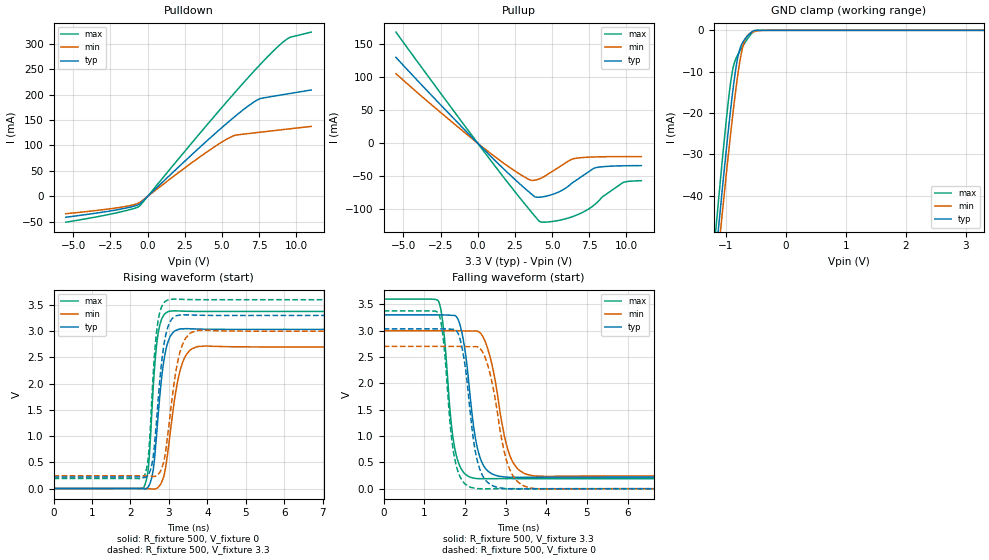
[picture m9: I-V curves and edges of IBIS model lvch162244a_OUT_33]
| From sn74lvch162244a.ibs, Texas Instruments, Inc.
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[Model]   lvch162244a_OUT_33
Model_type  3-state
Enable   Active-Low
Vref =   0
Rref =   500
Cref =   50p
Vmeas =   1.5
| variable   typ   min   max
C_comp   4.77pF   4.07pF   5.92pF
| C_pullup   2.94pF   2.22pF   4.55pF
| C_pulldown   2.77pF   2.29pF   3.86pF
| C_tri-state   4.77pF   4.07pF   5.92pF
[Temperature Range]   40   100   -40
| Ambient temperature   25   85   -40
[Voltage range]   3.3   3   3.6
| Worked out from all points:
|   slope of the pulldown table from 0 to 0.495 V, typ, clamps not added: 35.7 ohm
|   slope of the pullup table from 0 to 0.495 V, typ, clamps not added: 43.8 ohm
|   GND clamp passes 1 mA (typ) near -0.61 V on its own axis
|   rising waveform, R_fixture 500, V_fixture 0: 20-80 % time 236ps typ, 319ps min, 179ps max; typ from 0 V to 3.03 V
|   falling waveform, R_fixture 500, V_fixture 3.3: 20-80 % time 298ps typ, 400ps min, 236ps max; typ from 3.3 V to 0.22 V
|   rising waveform, R_fixture 500, V_fixture 3.3: 20-80 % time 234ps typ, 308ps min, 176ps max; typ from 0.22 V to 3.3 V
|   falling waveform, R_fixture 500, V_fixture 0: 20-80 % time 297ps typ, 396ps min, 237ps max; typ from 3.04 V to 0 V
[GND Clamp]
| lvch162244a_OUT_33
|   Voltage   I(typ)   I(min)   I(max)
-5.5V     -768.1mA   -753.5mA   -792mA
-1.18V    -56.86mA   -62.13mA   -50.54mA
-1.15V    -52.28mA   -57.69mA   -45.76mA
-1.1V     -44.75mA   -50.35mA   -37.9mA
-1.075V   -41.03mA   -46.73mA   -34.04mA
-955mV    -23.91mA   -29.87mA   -16.84mA
-885mV    -14.93mA   -20.68mA   -9.567mA
-810mV    -7.325mA   -11.87mA   -6.191mA
-745mV    -3.716mA   -5.877mA   -4.504mA
-610mV    -937.7uA   -884.1uA   -1.502mA
-470mV    -8.737uA   -130.2uA   -12.48uA
3.3V      64.68pA    54.59nA    -2.347nA
[Pulldown]
| lvch162244a_OUT_33
|   Voltage   I(typ)   I(min)   I(max)
-5.5V     -40.97mA   -34.05mA   -50.7mA
-1.905V   -25.55mA   -21.78mA   -31.11mA
-545mV    -15.11mA   -12.05mA   -19.05mA
2.915V    80.44mA    64.9mA     103.1mA
5.015V    135.8mA    107.1mA    175.4mA
5.895V    157.6mA    120.2mA    205mA
7.085V    184.2mA    124.5mA    243.9mA
7.645V    192.8mA    126.4mA    261.5mA
8.665V    197.8mA    129.8mA    291.7mA
9.36V     201.2mA    132.1mA    308.9mA
9.625V    202.5mA    133mA      313mA
11V       209.1mA    137.5mA    322.8mA
[Pullup]
| lvch162244a_OUT_33
|   Voltage   I(typ)   I(min)   I(max)
-5.5V     130.3mA    105.5mA    168.7mA
-1.46V    33.96mA    27.14mA    44.29mA
1.58V     -35.43mA   -27.59mA   -46.97mA
3.45V     -74.05mA   -55.08mA   -100.1mA
3.84V     -81.3mA    -56.09mA   -110.8mA
4.145V    -81.92mA   -54.11mA   -118.5mA
5.41V     -74.33mA   -37.07mA   -117.3mA
6.47V     -58.44mA   -23.37mA   -110.6mA
7.93V     -37.15mA   -20.8mA    -91.9mA
8.355V    -35.73mA   -20.57mA   -81.85mA
9.75V     -34.25mA   -20.26mA   -59.96mA
11V       -34.01mA   -20.24mA   -56.83mA
[Ramp]
| lvch162244a_OUT_33
| variable   typ   min   max
dV/dt_r   1.83/2.46E-10   1.63/3.32E-10   2.03/1.82E-10
dV/dt_f   1.85/3.08E-10   1.66/4.10E-10   2.05/2.40E-10
R_load = 500
[Rising Waveform]
| lvch162244a_OUT_33
R_fixture =   500
C_fixture =   0
L_fixture =   0
V_fixture =   0
V_fixture_min = 0
V_fixture_max = 0
|   Time   V(typ)   V(min)   V(max)
0s        711.3pV    1.74nV     18.52nV
2.34ns    -5.624mV   153.9uV    14.28mV
2.47ns    41.8mV     -3.632mV   423.2mV
2.595ns   368.6mV    -11.87mV   1.956V
2.71ns    1.302V     16.22mV    2.907V
2.86ns    2.391V     214mV      3.297V
3.03ns    2.894V     1.036V     3.382V
3.33ns    3.045V     2.346V     3.383V
3.8ns     3.039V     2.711V     3.376V
40ns      3.034V     2.7V       3.376V
[Falling Waveform]
| lvch162244a_OUT_33
R_fixture =   500
C_fixture =   0
L_fixture =   0
V_fixture =   3.3
V_fixture_min = 3
V_fixture_max = 3.6
|   Time   V(typ)   V(min)   V(max)
0s        3.3V       3V         3.6V
1.345ns   3.3V       3V         3.566V
1.47ns    3.298V     3V         3.051V
1.76ns    3.288V     3V         724mV
1.98ns    2.73V      2.996V     296.9mV
2.28ns    861.9mV    2.996V     193.2mV
2.61ns    307.8mV    2.525V     190.4mV
3.12ns    218mV      599mV      191.3mV
3.715ns   217.2mV    242mV      191.1mV
40ns      219.9mV    241.7mV    190.9mV
[Rising Waveform]
| lvch162244a_OUT_33
R_fixture =   500
C_fixture =   0
L_fixture =   0
V_fixture =   3.3
V_fixture_min = 3
V_fixture_max = 3.6
|   Time   V(typ)   V(min)   V(max)
0s        219.8mV    241.6mV    190.9mV
2.34ns    214.1mV    241.7mV    205.9mV
2.465ns   258.8mV    238mV      596.8mV
2.59ns    600.3mV    230mV      2.155V
2.705ns   1.542V     258mV      3.133V
2.855ns   2.664V     480.3mV    3.523V
3.025ns   3.167V     1.361V     3.607V
3.315ns   3.311V     2.664V     3.607V
3.775ns   3.304V     3.015V     3.6V
40ns      3.3V       3V         3.6V
[Falling Waveform]
| lvch162244a_OUT_33
R_fixture =   500
C_fixture =   0
L_fixture =   0
V_fixture =   0
V_fixture_min = 0
V_fixture_max = 0
|   Time   V(typ)   V(min)   V(max)
0s        3.035V     2.702V     3.376V
1.345ns   3.035V     2.702V     3.342V
1.465ns   3.034V     2.702V     2.855V
1.755ns   3.024V     2.701V     540.5mV
1.965ns   2.521V     2.699V     122.3mV
2.285ns   593.1mV    2.699V     3.016mV
2.595ns   96.66mV    2.251V     -734.4uV
3.085ns   -1.321mV   396.4mV    434.6uV
3.725ns   -2.873mV   197uV      139.2uV
40ns      17.73uV    29.56uV    5.191uV
